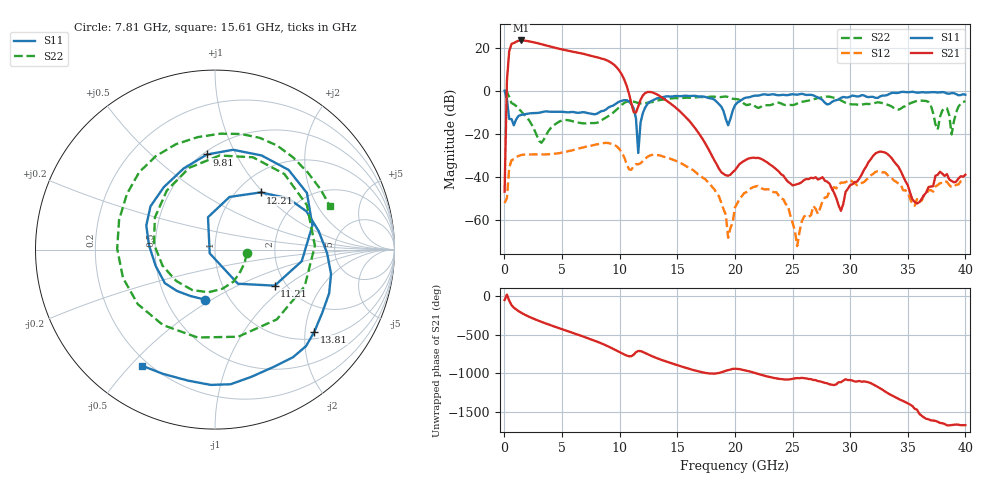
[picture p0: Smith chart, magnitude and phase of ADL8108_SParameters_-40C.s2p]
! Analog Devices, Inc.
! Device:	ADL8108 SN8565
! Description:	"GaAs, pHEMT, MMIC, Low Noise Amplifier, 1.5 GHz to 6 GHz"
! Conditions:	Vdd = 5.0 V
!		Idq = 90 mA
!  Rbias = 1270 Ohm
!		Pin = -25 dBm
!		Operating Temperature = -40 C (at package bottom)
! Board loss de-embedded from S21 magnitude.  All other RF measurements reference to RF coaxial connector.
! Frequency (GHz)	S11_Mag (dB)	S11_Phase (deg)	S21_Mag (dB)	S21_Phase (deg)	S12_Mag (dB)	S12_Phase (deg)	S22_Mag (dB)	S22_Phase (deg)
#  GHZ  S  DB  R 50
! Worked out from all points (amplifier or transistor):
!   201 points, 10 MHz to 40 GHz, reference 50 ohm
!   highest |S21| = 23.3 dB at 1.41 GHz (marker M1)
!   |S21| within 3 dB of that: 526.2 MHz to 4.118 GHz (3.592 GHz wide, 155 % of centre)
!   unconditionally stable (mu >= 1): 206.9 MHz to end of sweep
!   at 6.61 GHz: K = 1.37, MAG = 18.3 dB, |S12| = -26.5 dB
!   at 20 GHz: K = 8185.72, MAG = -33.5 dB, |S12| = -54.1 dB
!   at 40 GHz: K = 1228.39, MAG = -32.6 dB, |S12| = -41.5 dB
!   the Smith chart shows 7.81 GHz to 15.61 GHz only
!   S11 on the Smith chart (normalised r, x): 7.81 GHz: 0.77, -0.46; 9.81 GHz: 0.52, +0.77; 11.21 GHz: 1.75, -0.83; 12.21 GHz: 1.27, +0.97; 13.81 GHz: 1.19, -2.24; 15.61 GHz: 0.17, -0.54
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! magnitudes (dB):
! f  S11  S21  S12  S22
! 10 MHz  0.0  -46.8  -52.0  0.0
! 210 MHz  -3.9  4.5  -49.8  -0.4
! 410 MHz  -13.1  18.3  -35.6  -2.9
! 1.41 GHz  -11.3  23.3  -29.8  -9.4
! 6.81 GHz  -9.9  17.1  -26.3  -15.1
! 7.81 GHz  -10.9  15.7  -25.0  -15.0
! 9.81 GHz  -5.5  10.4  -26.1  -8.4
! 11.21 GHz  -8.2  -9.9  -34.9  -5.1
! 11.61 GHz  -28.9  -7.3  -34.1  -5.7
! 12.21 GHz  -7.8  -1.1  -31.5  -5.8
! 13.41 GHz  -3.3  -2.3  -29.9  -4.4
! 13.81 GHz  -2.9  -3.7  -30.6  -4.1
! 15.61 GHz  -2.3  -11.6  -34.5  -3.3
! 19.41 GHz  -16.0  -39.4  -68.2  -2.9
! 20.2 GHz  -5.6  -35.4  -52.2  -3.9
! 23.6 GHz  -2.0  -36.5  -47.0  -5.6
! 25.4 GHz  -1.9  -43.3  -72.0  -6.0
! 26.8 GHz  -2.1  -40.6  -53.4  -4.0
! 29.2 GHz  -3.3  -55.6  -42.5  -4.5
! 33.4 GHz  -1.5  -30.1  -40.0  -6.8
! 35.8 GHz  -0.9  -52.2  -50.2  -4.7
! 40 GHz  -1.9  -38.9  -41.5  -4.8
